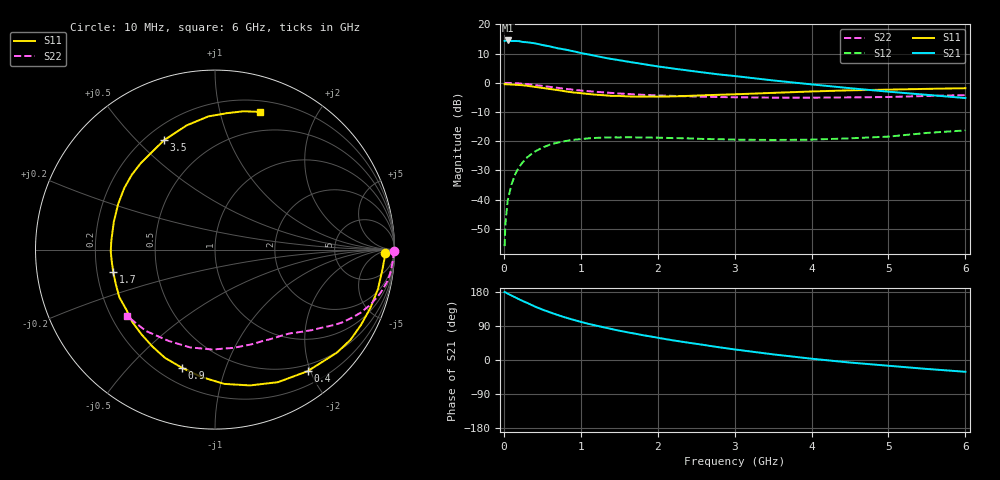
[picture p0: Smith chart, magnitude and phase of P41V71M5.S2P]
! SIEMENS Small Signal Semiconductors
! BFP182
! Si NPN RF Bipolar Junction Transistor in SOT143
! VCE = 1.75 V  IC = 1.5 mA
! Common Emitter S-Parameters:  March  1996
# GHz  S  MA  R  50
!  f  S11  S21  S12  S22
! GHz  MAG  ANG  MAG  ANG  MAG  ANG  MAG  ANG
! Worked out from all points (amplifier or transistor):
!   36 points, 10 MHz to 6 GHz, reference 50 ohm
!   highest |S21| = 14.5 dB at 50 MHz (marker M1)
!   |S21| within 3 dB of that: start of sweep to 771.9 MHz
!   unconditionally stable (mu >= 1): 2.375 GHz to end of sweep
!   at 250 MHz: K = 0.11, MSG = 20.5 dB, |S12| = -27.1 dB
!   at 1.4 GHz: K = 0.61, MSG = 13.4 dB, |S12| = -18.7 dB
!   at 6 GHz: K = 1.04, MAG = 4.3 dB, |S12| = -16.3 dB
!   S11 on the Smith chart (normalised r, x): 10 MHz: 31, -11; 400 MHz: 0.40, -1.95; 900 MHz: 0.29, -0.72; 1.7 GHz: 0.27, -0.10; 3.5 GHz: 0.27, +0.60; 6 GHz: 0.30, +1.33
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0.01  0.9446 -1.2  5.202 179.4  0.0016 86.5  0.9976 -0.5
0.02  0.9463 -2.7  5.258 178.7  0.0038 89.2  0.9921 -1.0
0.05  0.939 -7.1  5.299 175.0  0.0097 86.3  0.9949 -2.6
0.1  0.9341 -13.6  5.187 170.1  0.0182 81.5  0.9891 -5.3
0.15  0.9248 -20.5  5.195 165.1  0.0278 77.2  0.985 -7.9
0.2  0.9155 -27.2  5.154 160.0  0.0363 74.2  0.9759 -10.4
0.3  0.8894 -40.2  4.938 151.0  0.0525 66.3  0.9499 -15.2
0.4  0.8516 -52.7  4.744 141.5  0.0661 59.4  0.9181 -19.6
0.5  0.8177 -64.6  4.434 133.1  0.0776 52.1  0.8837 -23.5
0.6  0.7814 -75.6  4.183 125.8  0.0876 46.6  0.8507 -26.6
0.7  0.7499 -86.1  3.894 118.8  0.0947 41.9  0.8197 -29.5
0.8  0.7135 -96.2  3.697 112.2  0.1008 37.0  0.7894 -32.0
0.9  0.6836 -105.6  3.475 106.3  0.1057 33.3  0.7611 -34.2
1.1  0.6428 -122.9  3.057 95.4  0.112 26.6  0.7171 -38.1
1.4  0.5966 -146.0  2.553 81.8  0.1164 18.3  0.6704 -43.0
1.7  0.5808 -167.5  2.203 69.7  0.1162 13.2  0.6319 -47.4
2.2  0.5846 164.6  1.753 51.8  0.1131 7.5  0.5967 -54.9
2.8  0.6235 138.0  1.388 33.5  0.1082 5.2  0.5698 -65.2
3.5  0.6722 115.1  1.097 14.9  0.1051 6.4  0.5567 -79.7
4.5  0.7429 92.9  0.808 -6.7  0.1121 11.8  0.5623 -104.2
5.5  0.7871 78.3  0.622 -23.6  0.1387 15.4  0.5947 -130.4
6  0.8071 71.9  0.548 -31.1  0.1532 13.2  0.6148 -143.2
